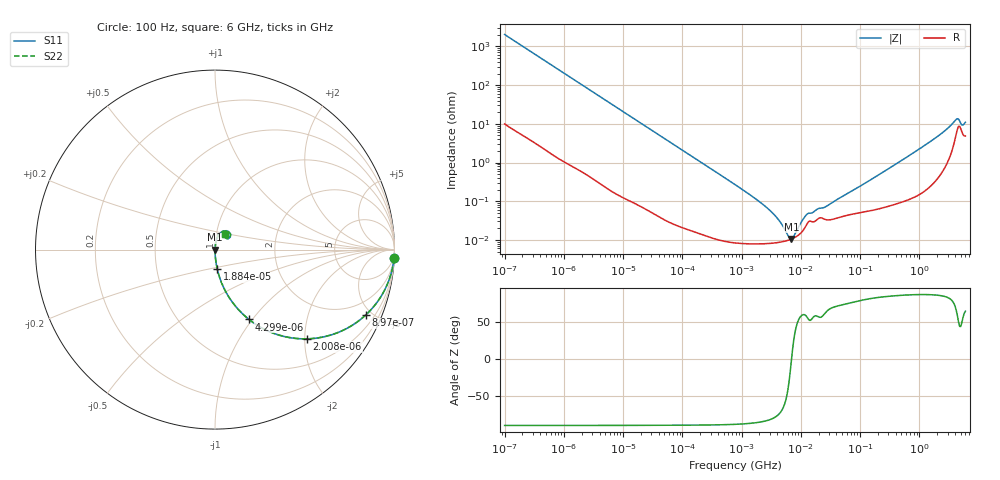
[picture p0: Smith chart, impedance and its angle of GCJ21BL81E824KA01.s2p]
!Murata Part Number: GCJ21BL81E824KA01
!These Parameters are Measured in Series Mode Connection
!Data Generated on Mar 13, 2026
!  o--ll--o
!Port1  Port2
!  o------o
!Operation Temp=25[degC], DC Bias Voltage=0[V]
!Freq. Start=100[Hz] Stop=6[GHz] 401[Steps]
# Hz S RI R 50
!Freq.(Hz) S11(Real) S11(Imag) S21(Real) S21(Imag) S12(Real) S12(Imag) S22(Real) S22(Imag)
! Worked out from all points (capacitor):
!   401 points, 100 Hz to 6 GHz, reference 50 ohm
!   read as one part in series: C = 778 nF near 109 Hz
!   lowest |Z| = 10.5 mohm at 6.949 MHz (marker M1)
!   series resonance near 6.981 MHz, so ESL is about 670 pH
!   S11 on the Smith chart (normalised r, x): 100 Hz: 1, -41; 897 Hz: 1.02, -4.58; 2.008 kHz: 1.01, -2.05; 4.299 kHz: 1.01, -0.96; 18.84 kHz: 1.00, -0.22; 6 GHz: 1.10, +0.20
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100  0.9974 -0.0488  0.00263 0.0488  0.00263 0.0488  0.9974 -0.0488
401  0.9624 -0.1878  0.0376 0.1878  0.0376 0.1878  0.9624 -0.1878
897  0.8389 -0.3651  0.1611 0.3651  0.1611 0.3651  0.8389 -0.3651
2008  0.5131 -0.497  0.4869 0.497  0.4869 0.497  0.5131 -0.497
4299  0.1892 -0.3889  0.8108 0.3889  0.8108 0.3889  0.1892 -0.3889
8047  0.0634 -0.2408  0.9366 0.2408  0.9366 0.2408  0.0634 -0.2408
18841  0.0128 -0.1088  0.9872 0.1088  0.9872 0.1088  0.0128 -0.1088
40335  0.00306 -0.0515  0.9969 0.0515  0.9969 0.0515  0.00306 -0.0515
774597  9.06e-05 -0.00269  0.9999 0.00269  0.9999 0.00269  9.06e-05 -0.00269
3103719  8.16e-05 -0.000547  0.9999 0.000547  0.9999 0.000547  8.16e-05 -0.000547
4440638  8.72e-05 -0.000284  0.9999 0.000284  0.9999 0.000284  8.72e-05 -0.000284
6353432  9.99e-05 -5.76e-05  0.9999 5.76e-05  0.9999 5.76e-05  9.99e-05 -5.76e-05
6948629  0.000105 -2.8e-06  0.9999 2.8e-06  0.9999 2.8e-06  0.000105 -2.8e-06
7599586  0.000112 5.25e-05  0.9999 -5.25e-05  0.9999 -5.25e-05  0.000112 5.25e-05
1.189169e7  0.000214 0.00035  0.9998 -0.00035  0.9998 -0.00035  0.000214 0.00035
1.555665e7  0.000294 0.000405  0.9997 -0.000405  0.9997 -0.000405  0.000294 0.000405
2.662322e7  0.000333 0.000647  0.9997 -0.000647  0.9997 -0.000647  0.000333 0.000647
3.124326e8  0.0008 0.00709  0.9992 -0.00709  0.9992 -0.00709  0.0008 0.00709
1.791126e9  0.00471 0.0407  0.9953 -0.0407  0.9953 -0.0407  0.00471 0.0407
4.009986e9  0.0497 0.1042  0.9503 -0.1042  0.9503 -0.1042  0.0497 0.1042
5.245841e9  0.0619 0.0624  0.9381 -0.0624  0.9381 -0.0624  0.0619 0.0624
6e9  0.0546 0.0889  0.9454 -0.0889  0.9454 -0.0889  0.0546 0.0889
